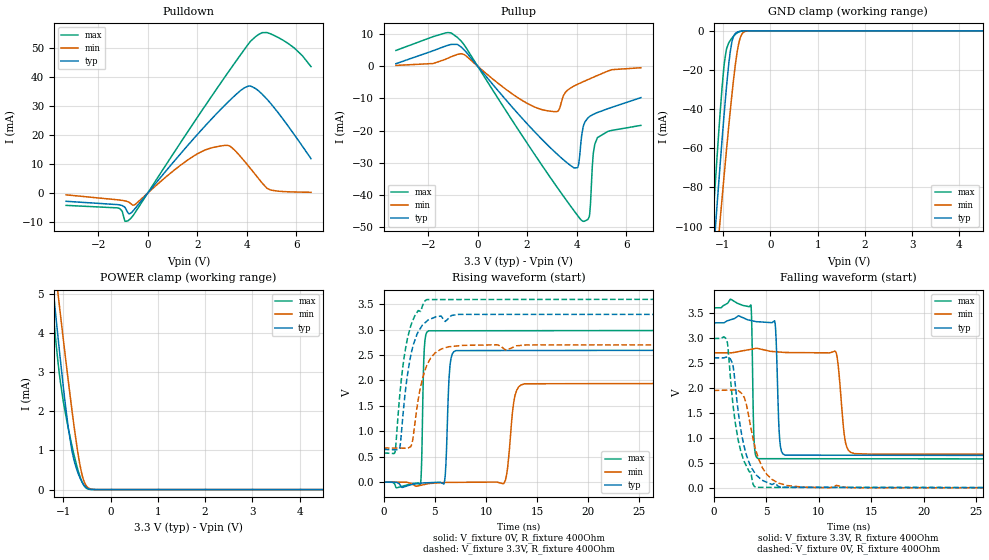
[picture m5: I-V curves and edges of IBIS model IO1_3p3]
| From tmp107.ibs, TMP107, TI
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|   Model
[Model]   IO1_3p3
Model_type   I/O
Polarity   Non-Inverting
Enable   Active-Low
Vinl = 0.99
Vinh = 2.31
Vmeas = 1.65
Vref = 0
Cref = 1pF
Rref = 100000
|   typ   min   max
C_comp   1.027pF   0.994pF   1.056pF
[Voltage Range]   3.3   2.7   3.6
[Temperature Range]   25   125   -55
[Pullup Reference]   3.3   2.7   3.6
[Pulldown Reference]   0   0   0
[Power Clamp Reference]   3.3   2.7   3.6
[GND Clamp Reference]   0   0   0
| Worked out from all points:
|   slope of the pulldown table from 0 to 0.495 V, typ, clamps not added: 96.5 ohm
|   slope of the pullup table from 0 to 0.495 V, typ, clamps not added: 107 ohm
|   GND clamp passes 1 mA (typ) near -0.72 V on its own axis
|   POWER clamp passes 1 mA (typ) near -0.82 V on its own axis
|   falling waveform, V_fixture 3.3V, R_fixture 400Ohm: 20-80 % time 245ps typ, 498ps min, 154ps max; typ from 3.3 V to 0.643 V
|   rising waveform, V_fixture 0V, R_fixture 400Ohm: 20-80 % time 285ps typ, 536ps min, 185ps max; typ from 0 V to 2.6 V
|   rising waveform, V_fixture 3.3V, R_fixture 400Ohm: 20-80 % time 1.19ns typ, 1.21ns min, 1.19ns max; typ from 0.643 V to 3.3 V
|   falling waveform, V_fixture 0V, R_fixture 400Ohm: 20-80 % time 1.3ns typ, 1.46ns min, 1.26ns max; typ from 2.6 V to 0 V
[Pulldown]
|   Voltage   I(typ)   I(min)   I(max)
-3.3V     -2.842mA   -617.9uA   -4.247mA
-1.211V   -3.986mA   -2.336mA   -5.113mA
-914.1mV  -4.969mA   -2.703mA   -9.732mA
-755.7mV  -7.204mA   -3.175mA   -9.267mA
-518.1mV  -5.403mA   -3.978mA   -6.839mA
1.393V    14.19mA    10.01mA    18.21mA
2.511V    24.89mA    15.39mA    32.45mA
3.313V    31.89mA    16.18mA    42.35mA
4.046V    36.78mA    9.568mA    51.08mA
4.828V    32.26mA    1.619mA    55.26mA
5.917V    20.2mA     368.3uA    50.02mA
6.6V      11.84mA    257.3uA    43.55mA
[GND Clamp]
|   Voltage   I(typ)   I(min)   I(max)
-3.3V     -846.1mA   -753.8mA   -932.7mA
-1.32V    -153.1mA   -169.1mA   -136.9mA
-1.201V   -113.4mA   -135.4mA   -91.62mA
-1.181V   -106.8mA   -129.9mA   -84.24mA
-1.122V   -87.46mA   -113.3mA   -62.57mA
-1.073V   -71.65mA   -99.65mA   -45.33mA
-973.5mV  -41.5mA    -72.91mA   -16.55mA
-844.8mV  -10.16mA   -40.18mA   -4.811mA
-686.4mV  -540.1uA   -8.704mA   -851.6uA
-597.3mV  -98.55uA   -1.548mA   -142.6uA
-458.7mV  -4.036uA   -44.39uA   -3.246uA
6.6V      0A         0A         0A
[Pullup]
|   Voltage   I(typ)   I(min)   I(max)
-3.3V     769.3uA    225uA      4.88mA
-815.1mV  6.75mA     3.651mA    8.909mA
2.65V     -23.14mA   -13.61mA   -31.36mA
3.244V    -27.55mA   -13.98mA   -37.96mA
3.551V    -29.61mA   -8.118mA   -41.28mA
3.897V    -31.63mA   -6.186mA   -44.94mA
4.085V    -30.41mA   -5.475mA   -46.88mA
4.264V    -18.96mA   -4.847mA   -48.21mA
4.521V    -15.69mA   -3.972mA   -46.43mA
4.67V     -15.01mA   -3.475mA   -27.64mA
4.838V    -14.43mA   -2.916mA   -22.3mA
6.6V      -9.768mA   -496uA     -18.41mA
[POWER Clamp]
|   Voltage   I(typ)   I(min)   I(max)
-3.3V     31.68mA    29.28mA    35.71mA
-1.28V    5.915mA    6.809mA    5.409mA
-1.162V   4.483mA    5.539mA    3.842mA
-1.102V   3.786mA    4.911mA    3.156mA
-1.003V   2.669mA    3.879mA    2.279mA
-943.8mV  2.048mA    3.273mA    1.876mA
-815.1mV  981.8uA    2.014mA    1.111mA
-745.8mV  634.6uA    1.388mA    753.3uA
-646.8mV  301.1uA    628.9uA    333.3uA
-567.6mV  124.3uA    232.8uA    112.4uA
-488.4mV  32.91uA    61.82uA    19.86uA
6.6V      0A         0A         0A
[Ramp]
R_load = 400
|   typ   min   max
dV/dt_r   1.55918/2.81921e-10   1.16844/5.30605e-10   1.79224/1.83786e-10
dV/dt_f   1.59447/2.42795e-10   1.21733/4.97428e-10   1.81552/1.53155e-10
[Falling Waveform]
V_fixture = 3.3V
V_fixture_min = 2.7V
V_fixture_max = 3.6V
R_fixture = 400Ohm
C_fixture = 0F
|   Time   V(typ)   V(min)   V(max)
0s        3.3V       2.7V       3.6V
3.547ns   3.347V     2.771V     3.66V
3.855ns   3.332V     2.783V     955.8mV
4.261ns   3.321V     2.785V     583.5mV
5.821ns   3.338V     2.723V     583.2mV
6.293ns   976.4mV    2.715V     583.1mV
6.819ns   654.3mV    2.707V     583mV
11.62ns   653mV      2.728V     582mV
13.4ns    652.5mV    686.6mV    581.6mV
50ns      642.5mV    671.1mV    574.1mV
[Rising Waveform]
V_fixture = 0V
V_fixture_min = 0V
V_fixture_max = 0V
R_fixture = 400Ohm
C_fixture = 0F
|   Time   V(typ)   V(min)   V(max)
0s        130.4nV    196.7nV    101.6nV
3.583ns   -22.65mV   -64.56mV   -48.57mV
3.961ns   -15.94mV   -47.92mV   2.599V
4.393ns   -12.08mV   -28.94mV   2.977V
5.97ns    41.15mV    -7.222mV   2.977V
6.469ns   2.261V     -5.556mV   2.977V
7.065ns   2.587V     -4.678mV   2.978V
11.76ns   2.589V     -24.67mV   2.979V
13.8ns    2.589V     1.935V     2.979V
50ns      2.599V     1.947V     2.987V
[Rising Waveform]
V_fixture = 3.3V
V_fixture_min = 2.7V
V_fixture_max = 3.6V
R_fixture = 400Ohm
C_fixture = 0F
|   Time   V(typ)   V(min)   V(max)
0s        642.5mV    671.1mV    574.1mV
1.101ns   636.9mV    669.3mV    580.8mV
1.588ns   690.8mV    668.5mV    1.748V
2.149ns   1.844V     667.6mV    2.647V
2.644ns   2.487V     696.4mV    3.073V
3.55ns    3.013V     1.824V     3.362V
4.234ns   3.17V      2.306V     3.592V
5.569ns   3.266V     2.613V     3.592V
7.837ns   3.299V     2.691V     3.592V
50ns      3.3V       2.7V       3.6V
[Falling Waveform]
|Gnd
V_fixture = 0V
V_fixture_min = 0V
V_fixture_max = 0V
R_fixture = 400Ohm
C_fixture = 0F
|   Time   V(typ)   V(min)   V(max)
0s        2.599V     1.947V     2.987V
1.271ns   2.618V     1.954V     2.938V
1.777ns   2.502V     1.957V     1.804V
2.33ns    1.55V      1.944V     969.2mV
2.887ns   846.5mV    1.817V     539.3mV
4.043ns   262.2mV    739.9mV    9.624mV
4.703ns   144.9mV    384mV      9.486mV
5.569ns   66.2mV     168.8mV    9.304mV
8.486ns   11.08mV    14.55mV    8.693mV
50ns      313.6nV    461.9nV    230.6nV
